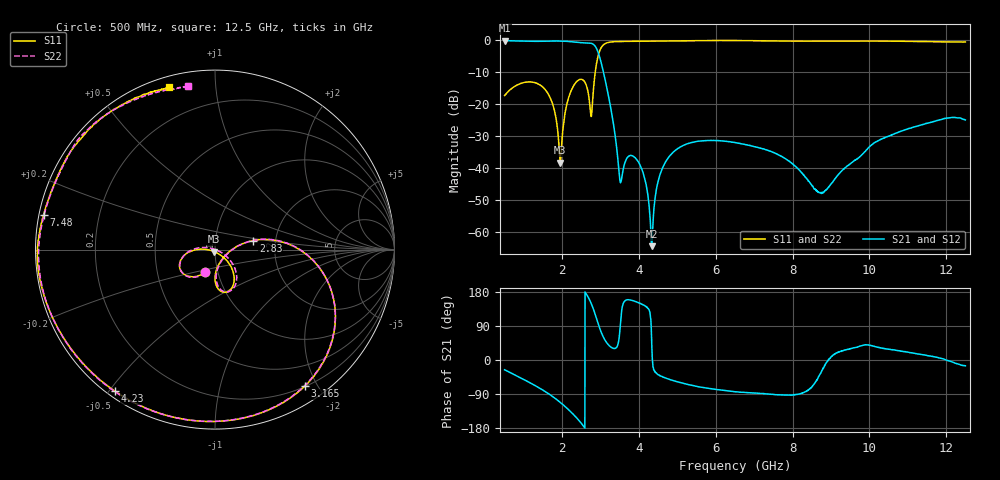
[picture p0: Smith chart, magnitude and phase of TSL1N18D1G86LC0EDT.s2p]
! TSL1N18D1G86LC0EDT  S-PARAMETER MODEL  ( General Type )
! Model Generated by TAIYO YUDEN Corporation (https://www.yuden.co.jp/en/)
! Version 1.0
! TAIYO YUDEN Control No. 20170328
! Copyright(c) 2017 TAIYO YUDEN CO.,LTD. All Rights Reserved.
! Products Name : Multilayer Ceramic Devices
! Characteristics :
!  Passband freq : 1710-2025MHz ( At Passband , Insertion Loss : 0.5dB , VSWR 2.0 ),
!  Attenuation : 27dB min at 3420-4050MHz , 30dB min at 5130-6075MHz , Impedance : 50 Ohm ,
!  Case Size : 1.6 x 0.8 / 0.063 x 0.031 [mm/inch] , Thickness : 0.65 / 0.026 [mm/inch]
!  (Conditions: Temperature = 25 degC , DC Bias Current/Voltage = 0A / 0V)
! External Node Assignments :
!  1  o---|-------|---o  2
!  |  LPF  |
! GND o---|-------|---o GND
! Frequency Range : 500MHz  -  12.5GHz  [ 2401 STEP ]
# MHZ S RI R 50
! Freq[MHz].  S11 Real  S11 Imag  S21 Real  S21 Imag  S12 Real  S12 Imag  S22 Real  S22 Imag
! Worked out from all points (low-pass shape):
!   2401 points, 500 MHz to 12.5 GHz, reference 50 ohm
!   highest |S21| = -0.11 dB at 500 MHz (marker M1); lowest = -64.3 dB at 4.33 GHz (marker M2)
!   |S21| within 3 dB of the highest: start of sweep to 2.914 GHz
!   lowest |S11| = -38.2 dB at 1.95 GHz (marker M3), VSWR 1.02, Z = 49.5 - j1.1 ohm
!   |S11| at or under -10 dB: start of sweep to 2.86 GHz
!   |S22| runs from -53.8 to -0.1 dB; largest |S21 - S12| = 0.0019
!   S11 on the Smith chart (normalised r, x): 500 MHz: 0.87, -0.22; 2.83 GHz: 1.53, +0.16; 3.165 GHz: 0.20, -1.83; 4.23 GHz: 0.02, -0.52; 7.48 GHz: 0.01, +0.10; 12.5 GHz: 0.05, +0.76
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500  -0.0551 -0.1255  0.8886 -0.4294  0.8873 -0.4308  -0.0531 -0.1269
1545  -0.1703 -0.0313  0.1271 -0.9563  0.1265 -0.9566  -0.1707 -0.0293
1795  -0.0811 0.00266  -0.1628 -0.958  -0.1632 -0.9578  -0.0792 0.0107
1950  -0.00507 -0.0111  -0.3617 -0.9015  -0.3623 -0.9012  0.000561 0.00196
2145  0.0808 -0.0809  -0.6057 -0.7435  -0.6064 -0.7433  0.0912 -0.0686
2500  0.0595 -0.2377  -0.8929 -0.2003  -0.8928 -0.1996  0.0719 -0.2354
2740  0.0315 -0.0651  -0.7992 0.4119  -0.7989 0.4128  0.034 -0.0664
2830  0.2129 0.0503  -0.5335 0.6544  -0.5328 0.6548  0.213 0.0509
2995  0.6642 -0.292  0.0981 0.4861  0.0983 0.4854  0.663 -0.2907
3165  0.4994 -0.7619  0.1261 0.125  0.1258 0.1249  0.4941 -0.7636
3510  0.0126 -0.9572  0.000178 0.00614  0.000164 0.00614  -0.00356 -0.957
3875  -0.3209 -0.9081  -0.0138 0.00626  -0.0138 0.00628  -0.3394 -0.9018
4230  -0.5585 -0.7887  -0.00281 0.00267  -0.0028 0.00263  -0.5711 -0.7818
4330  -0.6137 -0.7472  0.000384 0.000475  0.000366 0.000441  -0.6239 -0.7418
4500  -0.6976 -0.6733  0.00492 -0.00401  0.00495 -0.00393  -0.7034 -0.6703
5125  -0.8971 -0.3963  0.0109 -0.0196  0.0107 -0.0195  -0.8933 -0.4039
6500  -0.9892 -0.000542  0.00278 -0.0251  0.00258 -0.025  -0.9801 0.0407
7480  -0.9552 0.1938  -0.000231 -0.0179  -0.000302 -0.018  -0.9192 0.2993
8500  -0.8805 0.4003  0.00175 -0.00512  0.0018 -0.00515  -0.8239 0.5092
8795  -0.8584 0.4492  0.00395 -0.00151  0.00394 -0.0016  -0.8037 0.548
10500  -0.656 0.7126  0.0281 0.0151  0.0281 0.0152  -0.6397 0.7288
12500  -0.2557 0.9044  0.055 -0.015  0.0549 -0.0153  -0.1506 0.9118
